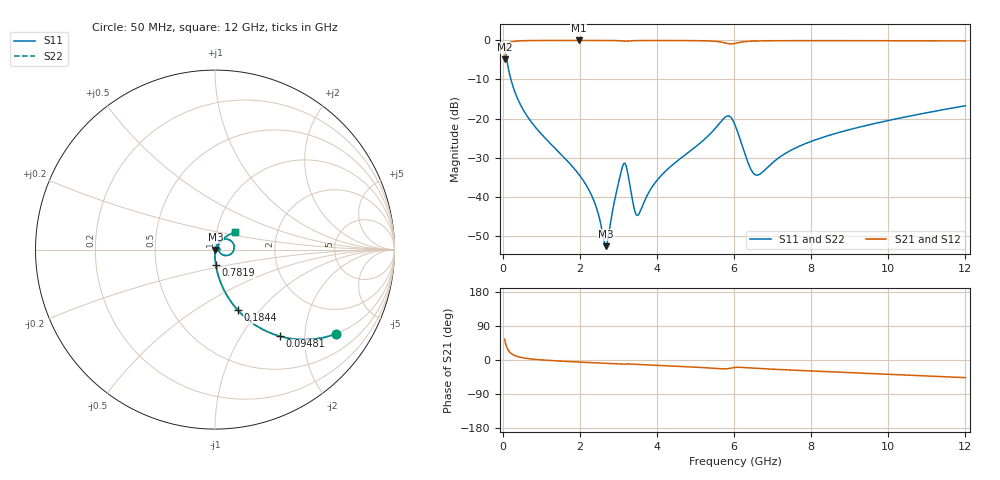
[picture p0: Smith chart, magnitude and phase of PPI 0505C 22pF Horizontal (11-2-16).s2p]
# MHz S MA R 50
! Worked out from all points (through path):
!   1601 points, 50 MHz to 12 GHz, reference 50 ohm
!   highest |S21| = -0.02 dB at 1.969 GHz (marker M1); lowest = -4.9 dB at 50 MHz (marker M2)
!   group delay of S21, straight-line fit = 12.2 ps
!   lowest |S11| = -52.7 dB at 2.679 GHz (marker M3), VSWR 1.00, Z = 50.2 - j0.0545 ohm
!   |S11| at or under -10 dB: 214.2 MHz to end of sweep
!   |S22| runs from -52.7 to -1.7 dB; largest |S21 - S12| = 0
!   S11 on the Smith chart (normalised r, x): 50 MHz: 0.99, -2.86; 94.81 MHz: 0.99, -1.51; 184.4 MHz: 0.99, -0.77; 781.9 MHz: 0.99, -0.17; 12 GHz: 1.22, +0.24
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50  0.8205 -35.0  0.5714 55.0  0.5714 55.0  0.8205 -35.0
94.8125  0.6033 -53.2  0.7972 36.8  0.7972 36.8  0.6033 -53.2
184.4375  0.3615 -69.3  0.9319 20.6  0.9319 20.6  0.3615 -69.3
415.9688  0.1668 -81.5  0.9853 8.2  0.9853 8.2  0.1668 -81.5
781.9375  0.08518 -87.1  0.9954 2.3  0.9954 2.3  0.08518 -87.1
1969.469  0.01947 -91.2  0.9983 -5.4  0.9983 -5.4  0.01947 -91.2
2044.156  0.01735 -90.9  0.9983 -5.8  0.9983 -5.8  0.01735 -90.9
2380.25  0.008503 -85.8  0.9981 -7.4  0.9981 -7.4  0.008503 -85.8
2679  0.002324 -13.5  0.9975 -8.8  0.9975 -8.8  0.002324 -13.5
3000.156  0.01479 47.2  0.9918 -10.6  0.9918 -10.6  0.01479 47.2
3134.594  0.02619 16.4  0.9765 -11.0  0.9765 -11.0  0.02619 16.4
3216.75  0.02307 -17.0  0.9769 -10.5  0.9769 -10.5  0.02307 -17.0
3396  0.007568 -21.3  0.9923 -11.1  0.9923 -11.1  0.007568 -21.3
3485.625  0.005743 9.8  0.9944 -11.6  0.9944 -11.6  0.005743 9.8
4038.312  0.017 65.0  0.9964 -14.2  0.9964 -14.2  0.017 65.0
5778.531  0.1048 23.6  0.9251 -23.3  0.9251 -23.3  0.1048 23.6
6025  0.08292 -21.5  0.9167 -19.5  0.9167 -19.5  0.08292 -21.5
6390.969  0.02509 -23.4  0.9745 -20.8  0.9745 -20.8  0.02509 -23.4
6577.688  0.01888 6.7  0.983 -22.0  0.983 -22.0  0.01888 6.7
8019.156  0.0514 54.8  0.9926 -28.9  0.9926 -28.9  0.0514 54.8
10013.31  0.09462 49.5  0.9901 -37.6  0.9901 -37.6  0.09462 49.5
12000  0.1458 41.5  0.9836 -46.6  0.9836 -46.6  0.1458 41.5
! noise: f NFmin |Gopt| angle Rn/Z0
50  0.0003961  0.868  1.001  0.0006451
1372  0.004042  0.678  4.718  0.002421
2701  0.008139  0.6847  8.915  0.004977
4031  0.01141  0.6689  13.19  0.006537
5360  0.02719  0.8018  17.48  0.02781
6682  0.03028  0.7822  21.78  0.02752
8012  0.02127  0.6574  25.73  0.01129
9341  0.02131  0.6154  29.57  0.009669
1.067e+04  0.02272  0.5973  33.32  0.009576
1.2e+04  0.02463  0.5897  36.96  0.009956
